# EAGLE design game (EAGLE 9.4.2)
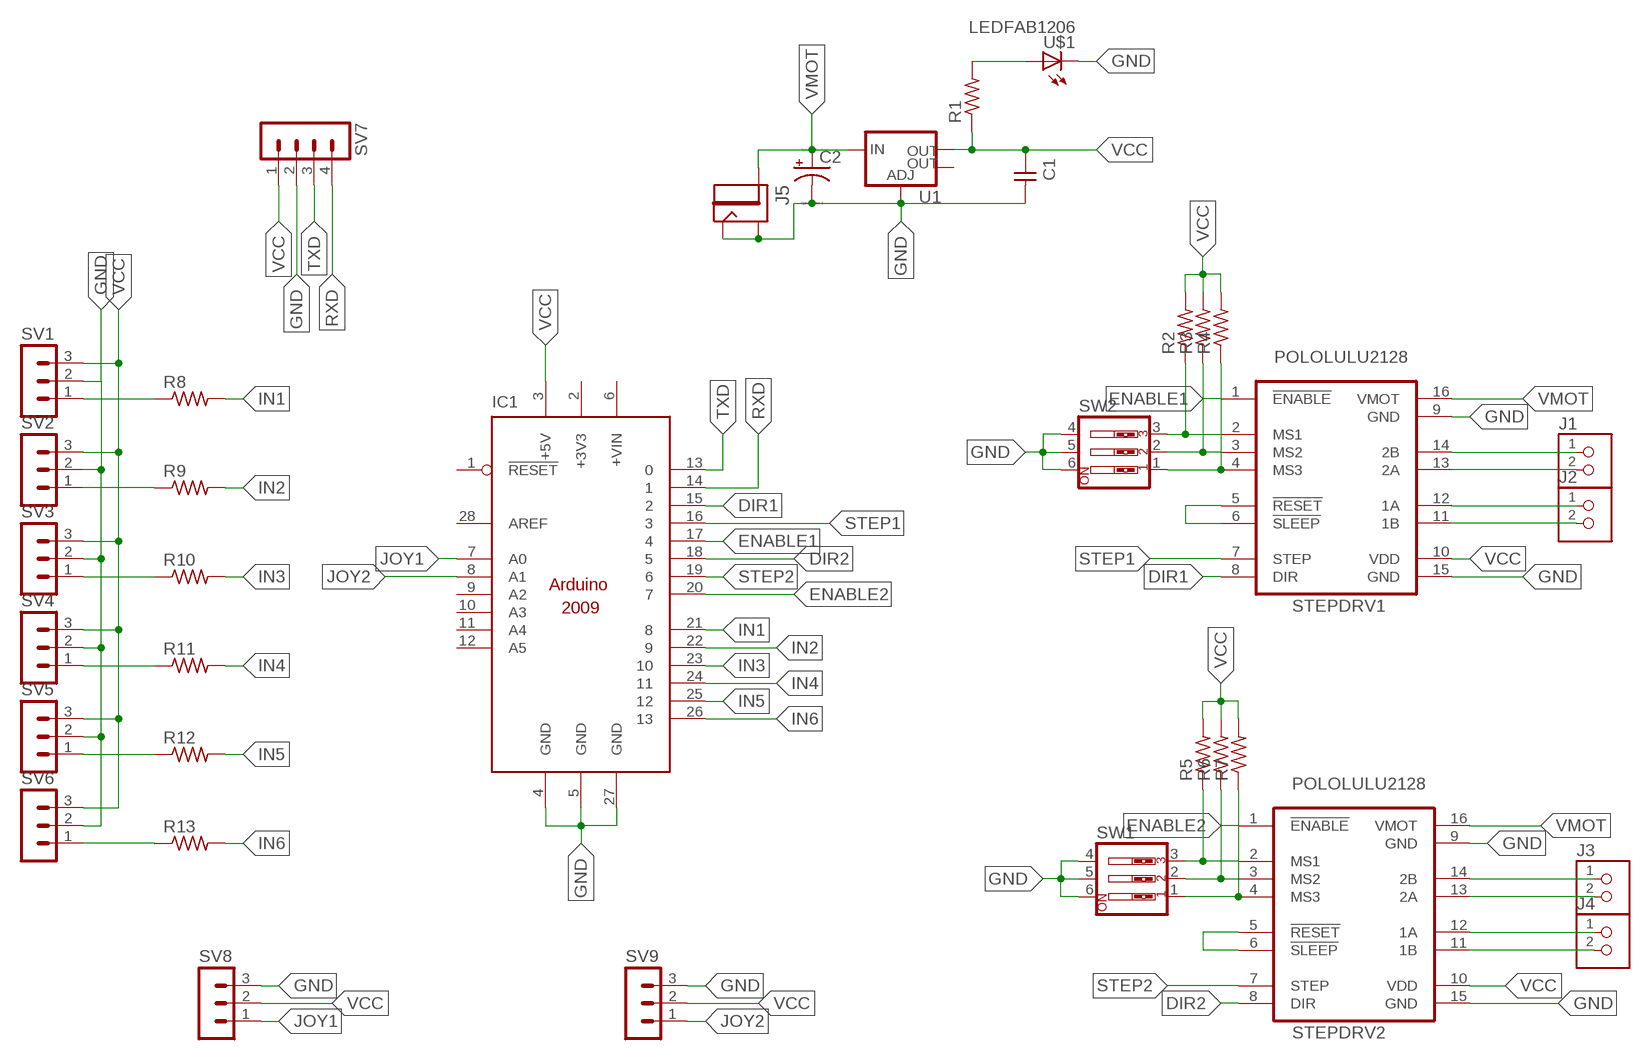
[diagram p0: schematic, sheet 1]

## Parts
C1  CAP-UNPOLARIZEDFAB  [C1206FAB]
C2  CPOL-USE1.8-4  [E1,8-4]
IC1  ARDUINO2009_10  [ARDUINO2009]
J1  TERM-1X02-ADAFRUIT  [3.5MMTERM]
J2  TERM-1X02-ADAFRUIT  [3.5MMTERM]
J3  TERM-1X02-ADAFRUIT  [3.5MMTERM]
J4  TERM-1X02-ADAFRUIT  [3.5MMTERM]
J5  JACK2.1MM  [JACK_2.1MM]
R1  RES-US1206FAB  [R1206FAB]
R2  RES-US1206FAB  [R1206FAB]
R3  RES-US1206FAB  [R1206FAB]
R4  RES-US1206FAB  [R1206FAB]
R5  RES-US1206FAB  [R1206FAB]
R6  RES-US1206FAB  [R1206FAB]
R7  RES-US1206FAB  [R1206FAB]
R8  RES-US1206FAB  [R1206FAB]
R9  RES-US1206FAB  [R1206FAB]
R10  RES-US1206FAB  [R1206FAB]
R11  RES-US1206FAB  [R1206FAB]
R12  RES-US1206FAB  [R1206FAB]
R13  RES-US1206FAB  [R1206FAB]
STEPDRV1  POLOLULU2128  [POLOLULU2128]
STEPDRV2  POLOLULU2128  [POLOLULU2128]
SV1  MA03-1  [MA03-1]
SV2  MA03-1  [MA03-1]
SV3  MA03-1  [MA03-1]
SV4  MA03-1  [MA03-1]
SV5  MA03-1  [MA03-1]
SV6  MA03-1  [MA03-1]
SV7  MA04-1  [MA04-1]
SV8  MA03-1  [MA03-1]
SV9  MA03-1  [MA03-1]
SW1  SW_DIP-3  [EDG-03]
SW2  SW_DIP-3  [EDG-03]
U1  V_REG_LM1117SOT223  [SOT223]
U$1  LEDFAB1206  [LED1206FAB]

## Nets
DIR1: IC1.15 STEPDRV1.8(DIR)
DIR2: IC1.18 STEPDRV2.8(DIR)
ENABLE1: IC1.17 STEPDRV1.1(!ENABLE)
ENABLE2: IC1.20 STEPDRV2.1(!ENABLE)
GND: C1.2 C2.- IC1.4(GND) IC1.5(GND) IC1.27(GND) J5.CONTACT J5.SHUNT STEPDRV1.9(GND) STEPDRV1.15(GND) STEPDRV2.9(GND) STEPDRV2.15(GND) SV1.2 SV2.2 SV3.2 SV4.2 SV5.2 SV6.2 SV7.2 SV8.3 SV9.3 SW1.4 SW1.5 SW1.6 SW2.4 SW2.5 SW2.6 U1.1(ADJ) U$1.2(C)
IN1: IC1.21 R8.2
IN2: IC1.22 R9.2
IN3: IC1.23 R10.2
IN4: IC1.24 R11.2
IN5: IC1.25 R12.2
IN6: IC1.26 R13.2
JOY1: IC1.7(A0) SV8.1
JOY2: IC1.8(A1) SV9.1
N$1: R2.1 STEPDRV1.2(MS1) SW2.3
N$2: STEPDRV1.5(!RESET) STEPDRV1.6(!SLEEP)
N$3: R8.1 SV1.1
N$4: R9.1 SV2.1
N$5: STEPDRV2.5(!RESET) STEPDRV2.6(!SLEEP)
N$6: R3.1 STEPDRV1.3(MS2) SW2.2
N$7: R4.1 STEPDRV1.4(MS3) SW2.1
N$9: J1.1 STEPDRV1.14(2B)
N$10: J1.2 STEPDRV1.13(2A)
N$11: J3.1 STEPDRV2.14(2B)
N$12: J3.2 STEPDRV2.13(2A)
N$13: J4.1 STEPDRV2.12(1A)
N$14: J4.2 STEPDRV2.11(1B)
N$15: R10.1 SV3.1
N$16: R11.1 SV4.1
N$17: J2.1 STEPDRV1.12(1A)
N$18: J2.2 STEPDRV1.11(1B)
N$19: R12.1 SV5.1
N$20: R13.1 SV6.1
N$24: R5.1 STEPDRV2.2(MS1) SW1.3
N$25: R6.1 STEPDRV2.3(MS2) SW1.2
N$26: R7.1 STEPDRV2.4(MS3) SW1.1
N$27: R1.2 U$1.1(A)
RXD: IC1.14 SV7.4
STEP1: IC1.16 STEPDRV1.7(STEP)
STEP2: IC1.19 STEPDRV2.7(STEP)
TXD: IC1.13 SV7.3
VCC: C1.1 IC1.3(+5V) R1.1 R2.2 R3.2 R4.2 R5.2 R6.2 R7.2 STEPDRV1.10(VDD) STEPDRV2.10(VDD) SV1.3 SV2.3 SV3.3 SV4.3 SV5.3 SV6.3 SV7.1 SV8.2 SV9.2 U1.2(OUT)
VMOT: C2.+ J5.PIN STEPDRV1.16(VMOT) STEPDRV2.16(VMOT) U1.3(IN)
Unconnected: IC1.1(!RESET) IC1.6(+VIN) IC1.9(A2) IC1.10(A3) IC1.11(A4) IC1.12(A5) IC1.28(AREF) U1.4(OUT)

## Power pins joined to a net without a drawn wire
+3V3: IC1.2(+3V3)

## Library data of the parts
C1 = fab:CAP-UNPOLARIZED
C2 = resistor:CPOL-US: POLARIZED CAPACITOR, American symbol
IC1 = arduino:ARDUINO2009_1: The Arduino Duemilanove ("2009") is a microcontroller board based on the ATmega168 or ATmega328. - 14 digital input/output pins (of which 6 can be used as PWM outputs) - 6 analog inputs, a 16 MHz crystal oscillator - USB connection - power jack - ISP header - reset button It contains everything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
J1-J4 = fab:TERM-1X02: 3.5mm terminal block, 2 positions ED555-2DS as found in the fablab inventory.
J5 = fab:JACK
R1-R13 = fab:RES-US: Resistor (US Symbol)
STEPDRV1 STEPDRV2 = stepper_drivers_etc:POLOLULU2128
SV1-SV6 SV8 SV9 = con-lstb:MA03-1: PIN HEADER; OC_FARNELL: unknown; OC_NEWARK: unknown
SV7 = con-lstb:MA04-1: PIN HEADER; OC_FARNELL: unknown; OC_NEWARK: unknown
SW1 SW2 = special:SW_DIP-3: DIP SWITCH
U1 = fab:V_REG_LM1117: Voltage Regulator LM1117 Standard adjustable voltage regulator but in SMD form. Spark Fun Electronics SKU : COM-00595; PROD_ID: VREG-08170
U$1 = fab:LED: LED

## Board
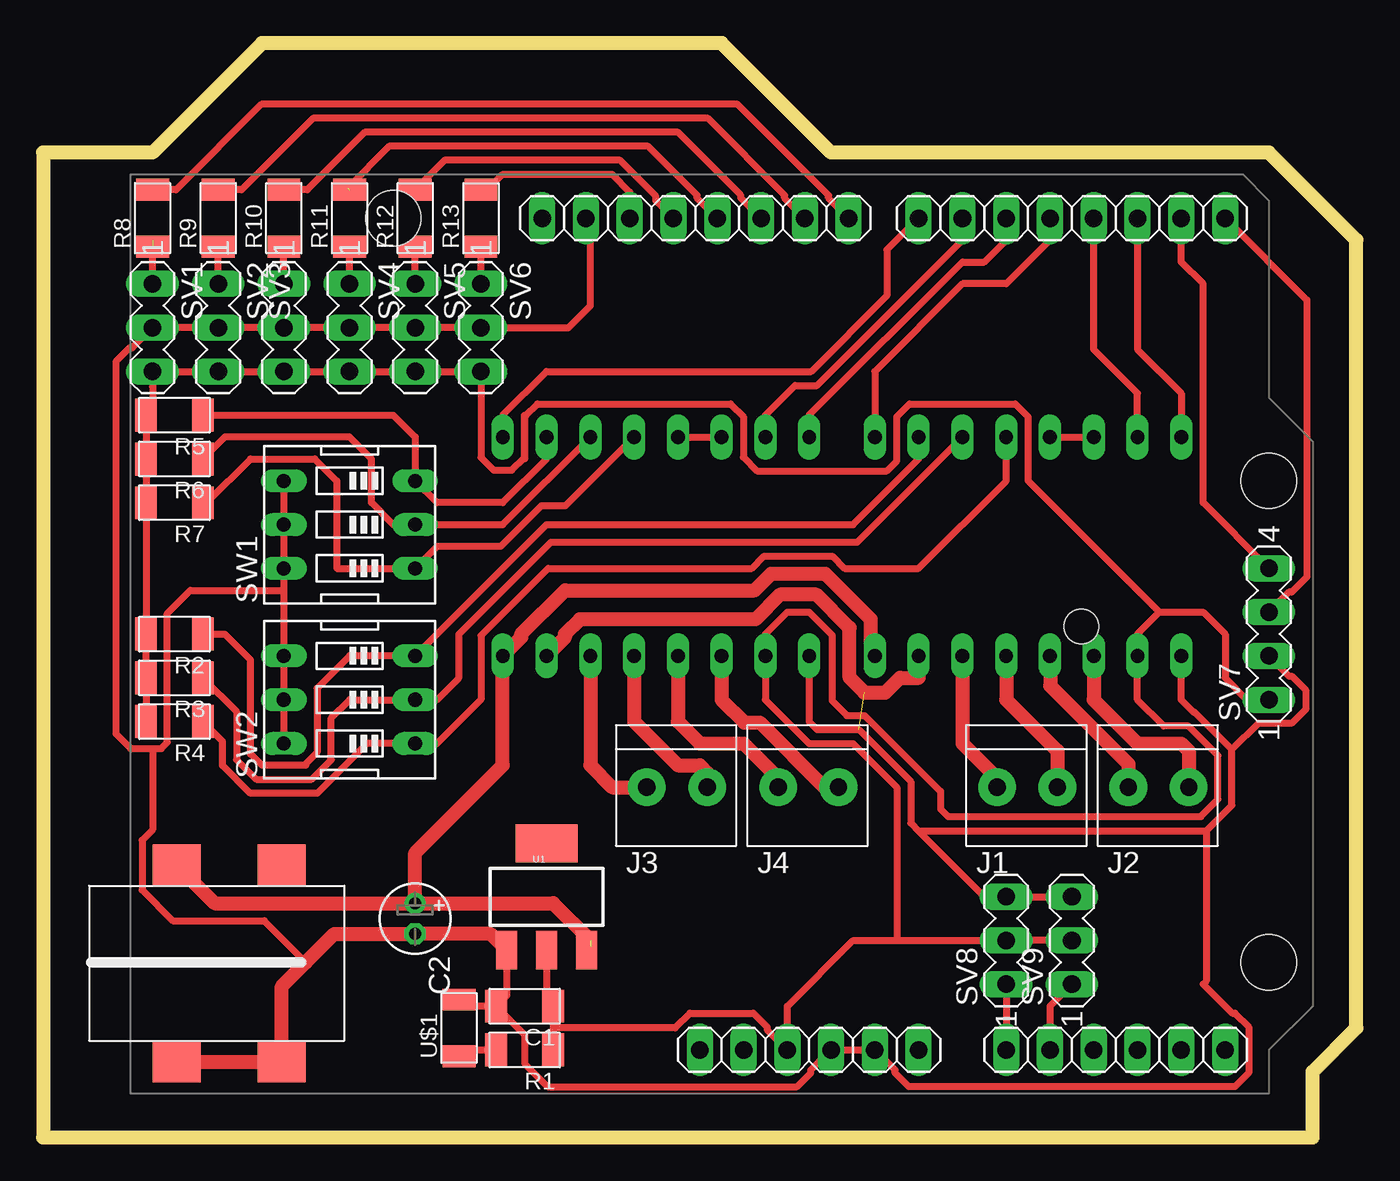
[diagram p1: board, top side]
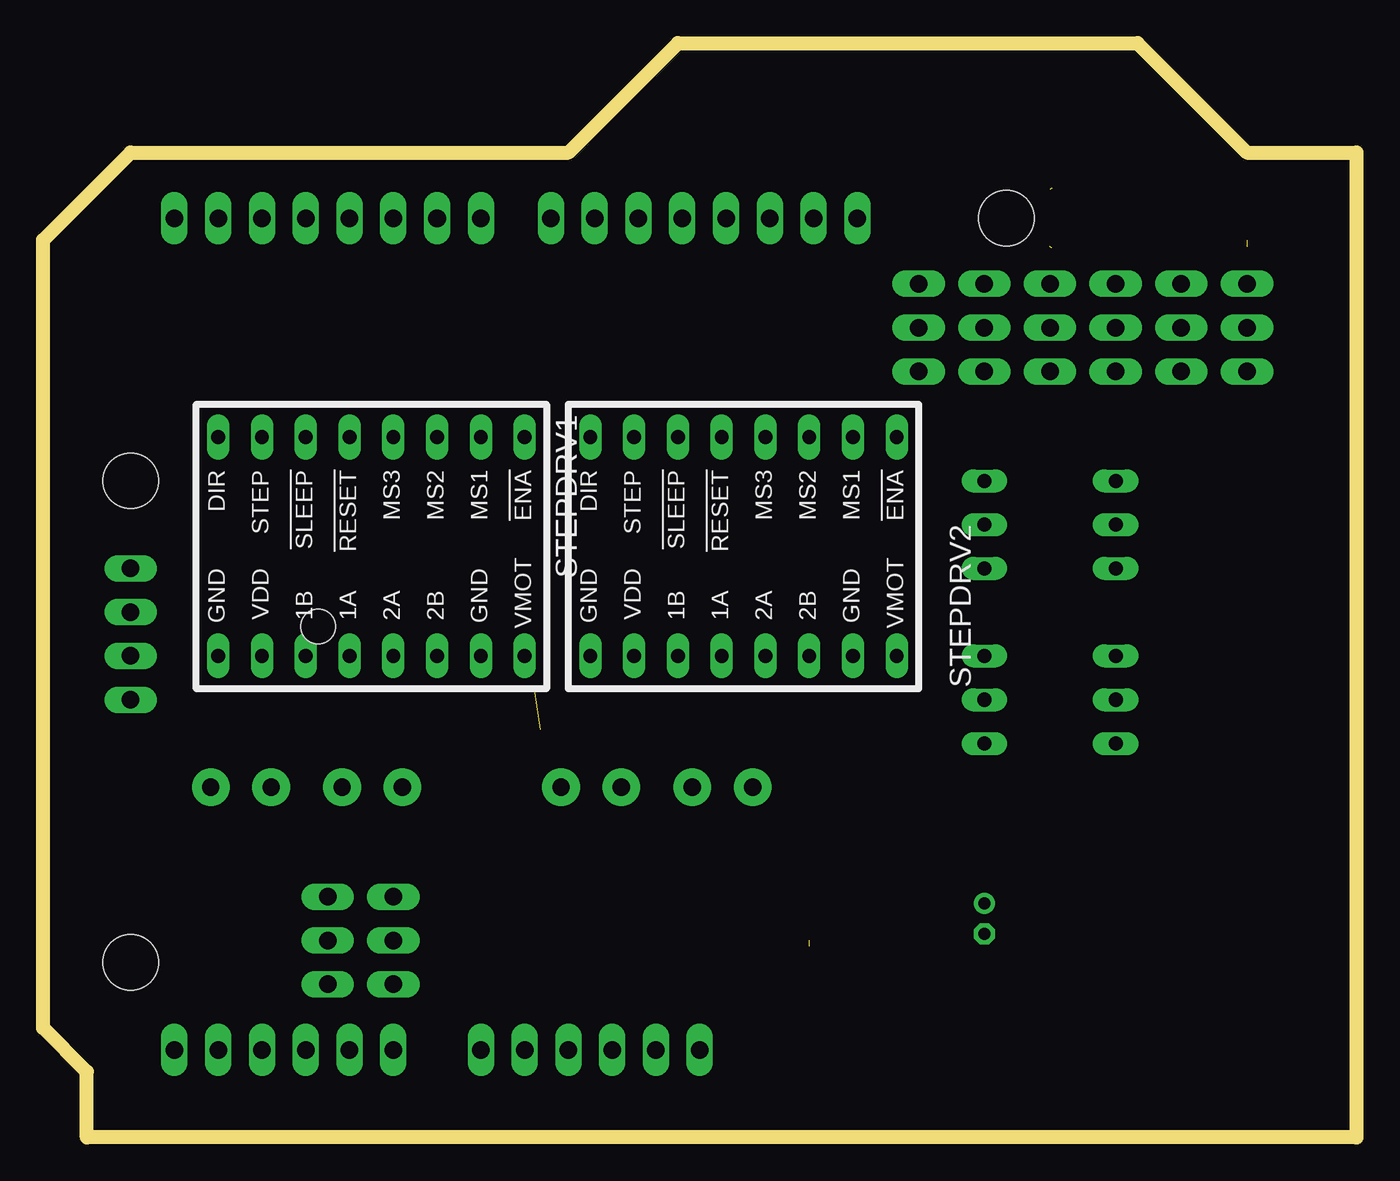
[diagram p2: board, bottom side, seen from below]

Size 76.2 x 63.5 mm. Coordinates in mm from the lower left corner, seen from the top.
Outline: 12.7,63.5 6.35,57.15 0,57.15 0,0 73.66,0 73.66,3.81 76.2,6.35 76.2,52.07 71.12,57.15 45.72,57.15 39.37,63.5 12.7,63.5
Copper layers (1*16): Top 0.035mm / dielectric 1.5mm / Bottom 0.035mm
Design rules "default *": minimum track width 16mil, minimum drill 0.35mm, track to track 16mil, track to pad 16mil, pad to pad 16mil, via to via 16mil, smd to smd 16mil, copper to edge 16mil, drill to drill 16mil, minimum pad ring 10mil, minimum via ring 8mil, stop-mask expansion 4mil, vias tented up to drill 0mil, thermal gap 10mil

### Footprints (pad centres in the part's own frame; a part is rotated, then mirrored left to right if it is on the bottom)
C1206FAB = smd 1.27 x 1.905: 1 -1.651,0; 2 1.651,0
E1,8-4 = drill 0.711 pad 1.168: + -0.889,0 | drill 0.711 pad 1.168 octagon: - 0.889,0
ARDUINO2009 = drill 1.016 long: 1 33.02,2.54; 2 35.56,2.54; 3 38.1,2.54; 4 40.64,2.54; 5 43.18,2.54; 6 45.72,2.54; 7 50.8,2.54; 8 53.34,2.54; 9 55.88,2.54; 10 58.42,2.54; 11 60.96,2.54; 12 63.5,2.54; 13 63.5,50.8; 14 60.96,50.8; 15 58.42,50.8; 16 55.88,50.8; 17 53.34,50.8; 18 50.8,50.8; 19 48.26,50.8; 20 45.72,50.8; 21 41.656,50.8; 22 39.116,50.8; 23 36.576,50.8; 24 34.036,50.8; 25 31.496,50.8; 26 28.956,50.8; 27 26.416,50.8; 28 23.876,50.8 | hole 3.2: 15.24,50.8; 66.04,35.56; 66.04,7.62 | hole 2: 55.17,27.114
3.5MMTERM = drill 1 pad 2.184: 1 1.8,0; 2 -1.7,0
JACK_2.1MM = smd 2.388 x 2.794: CONTACT 5.766,-2.413; PIN -5.639,-2.413; PIN1 -5.639,3.683; SHUNT 5.766,3.683
R1206FAB = smd 1.27 x 1.905: 1 -1.651,0; 2 1.651,0
POLOLULU2128 = drill 0.8 long: 1 -7.62,7.62; 2 -7.62,5.08; 3 -7.62,2.54; 4 -7.62,0; 5 -7.62,-2.54; 6 -7.62,-5.08; 7 -7.62,-7.62; 8 -7.62,-10.16; 9 5.08,-10.16; 10 5.08,-7.62; 11 5.08,-5.08; 12 5.08,-2.54; 13 5.08,0; 14 5.08,2.54; 15 5.08,5.08; 16 5.08,7.62
MA03-1 = drill 1.016 long: 1 -2.54,0; 2 0,0; 3 2.54,0
MA04-1 = drill 1.016 long: 1 -3.81,0; 2 -1.27,0; 3 1.27,0; 4 3.81,0
EDG-03 = drill 0.813 long: 1 -2.54,-3.81; 2 0,-3.81; 3 2.54,-3.81; 4 2.54,3.81; 5 0,3.81; 6 -2.54,3.81
SOT223 = smd 1.219 x 2.235: 1 -2.311,-3.099; 2 0,-3.099; 3 2.311,-3.099 | smd 3.6 x 2.2: 4 0,3.099
LED1206FAB = smd 1.27 x 1.905: 1 -1.651,0; 2 1.651,0

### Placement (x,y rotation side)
C1  27.94,7.62 180 top
C2  21.59,12.7 270 top
IC1  5.08,2.54 0 top
J1  57.15,20.32 180 top
J2  64.77,20.32 180 top
J3  36.83,20.32 180 top
J4  44.45,20.32 180 top
J5  10.16,10.16 270 top
R1  27.94,5.08 180 top
R2  7.62,29.21 180 top
R3  7.62,26.67 180 top
R4  7.62,24.13 180 top
R5  7.62,41.91 180 top
R6  7.62,39.37 180 top
R7  7.62,36.83 180 top
R8  6.35,53.34 90 top
R9  10.16,53.34 90 top
R10  13.97,53.34 90 top
R11  17.78,53.34 90 top
R12  21.59,53.34 90 top
R13  25.4,53.34 90 top
STEPDRV1  55.88,33.02 270 bottom
STEPDRV2  34.29,33.02 270 bottom
SV1  6.35,46.99 270 top
SV2  10.16,46.99 270 top
SV3  13.97,46.99 270 top
SV4  17.78,46.99 270 top
SV5  21.59,46.99 270 top
SV6  25.4,46.99 270 top
SV7  71.12,29.21 90 top
SV8  55.88,11.43 90 top
SV9  59.69,11.43 90 top
SW1  17.78,35.56 90 top
SW2  17.78,25.4 90 top
U1  29.21,13.97 0 top
U$1  24.13,6.35 90 top

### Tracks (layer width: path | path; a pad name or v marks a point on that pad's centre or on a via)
DIR1
  Top 0.406: STEPDRV1.8 66.04,43.18 63.5,45.72 IC1.15
DIR2
  Top 0.406: STEPDRV2.8 44.45,41.91 53.34,50.8 54.61,50.8 55.88,52.07 IC1.18
ENABLE1
  Top 0.406: IC1.17 58.42,52.07 55.88,49.53 53.34,49.53 48.26,44.45 STEPDRV1.1
ENABLE2
  Top 0.406: STEPDRV2.1 26.67,41.91 29.21,44.45 44.57,44.45 48.96,48.84 48.96,51.5 IC1.20
GND  (1 unrouted)
  Top 0.406: SV9.3 SV8.3 54.61,13.97 50.8,17.78 | 68.99,22.5 68.99,19.28 67.49,17.78 | 68.99,22.5 66.8,24.69 66.75,24.69 66.04,25.4 STEPDRV1.9 | U1.1 26.9,8.23 C1.2 | C1.2 24.51,7.62 U$1.2 | C1.2 27.94,5.97 27.94,4.28 29.27,2.95 43.75,2.95 44.55,3.75 44.55,3.91 IC1.4 IC1.5 49.43,3.91 49.43,3.75 50.23,2.95 69.15,2.95 69.95,3.75 69.95,6.41 69.15,7.21 68.99,7.21 67.31,8.89 67.49,9.07 67.49,17.78 | IC1.27 31.75,53.09 31.75,48.26 30.48,46.99 SV6.2 SV5.2 SV4.2 SV3.2 SV2.2 SV1.2 5.18,45.82 5.02,45.82 4.22,45.02 4.22,23.43 5.08,22.57 6.35,22.57 | 68.99,22.5 70.51,24.03 72.45,24.03 73.25,24.83 73.25,25.97 72.45,26.77 72.29,26.77 SV7.2 | 50.8,17.78 50.34,18.24 50.34,20.66 47.33,23.67 44.91,23.67 44.45,24.13 STEPDRV2.9 | 50.8,17.78 67.49,17.78 | SW1.4 SW1.6 | SW1.5 SW1.6 | SW2.6 SW2.5 SW2.4 13.97,31.75 | SW1.6 13.97,31.75 | 6.35,22.57 6.86,22.57 7.21,22.92 7.21,30.41 8.55,31.75 13.97,31.75 | 15.24,10.16 12.83,12.57 7.52,12.57 5.74,14.35 5.74,17.25 6.35,17.86 6.35,22.57
  Top 0.813: J5.CONTACT J5.SHUNT 13.84,8.76 15.24,10.16 16.89,11.81 C2.- 25.96,11.81 U1.1 | STEPDRV1.15 50.8,26.67 49.72,26.67 48.87,25.82 47.65,25.82 46.79,26.68 46.79,29.57 44.87,31.5 42.76,31.5 41.32,30.06 31.14,30.06 30.28,29.2 30.28,29.01 STEPDRV2.15
IN1
  Top 0.406: IC1.21 45.57,54.51 45.57,54.67 40.29,59.94 12.66,59.94 7.71,54.99 R8.2
IN2
  Top 0.406: IC1.22 43.03,54.51 43.03,54.67 38.57,59.13 15.66,59.13 11.52,54.99 R9.2
IN3
  Top 0.406: IC1.23 40.49,54.51 40.49,54.67 36.84,58.32 18.66,58.32 15.33,54.99 R10.2
IN4  (1 unrouted)
  Top 0.406: IC1.24 37.95,54.51 37.95,54.67 35.11,57.51 20.09,57.51 17.68,55.09
IN5
  Top 0.406: IC1.25 35.56,54.36 35.56,54.61 33.48,56.69 23.29,56.69 R12.2
IN6
  Top 0.406: R13.2 25.78,54.99 26.67,55.88 33.02,55.88 34.04,54.86 IC1.26
JOY1
  Top 0.406: SV8.1 IC1.7
JOY2
  Top 0.406: SV9.1 58.42,7.62 IC1.8
N$1
  Top 0.406: 8.89,29.21 R2.1 10.54,29.21 12.04,27.71 12.04,22.25 12.7,21.59 15.24,21.59 15.24,21.67 15.9,22.33 15.9,26.06 17.78,27.94 SW2.3 29.21,35.56 46.99,35.56 50.8,39.37 STEPDRV1.2
N$2
  Top 0.406: STEPDRV1.5 STEPDRV1.6
N$3  (1 unrouted)
  Top 0.406: SV1.1 6.35,52.07
N$4
  Top 0.406: SV2.1 R9.1
N$5
  Top 0.406: STEPDRV2.5 STEPDRV2.6
N$6
  Top 0.406: 9.27,26.58 R3.1 11.23,24.71 11.23,21.91 12.36,20.78 15.58,20.78 16.71,21.91 16.71,24.33 17.78,25.4 SW2.2 22.86,25.4 24.13,26.67 24.13,29.21 29.46,34.54 47.24,34.54 STEPDRV1.3
N$7
  Top 0.406: STEPDRV1.4 55.88,38.1 50.8,33.02 46.51,33.02 45.8,33.73 41.83,33.73 41.12,33.02 29.31,33.02 25.41,29.12 25.41,25.41 22.86,22.86 SW2.1 18.81,22.86 15.91,19.96 12.03,19.96 10.41,21.58 10.41,22.99 R4.1
N$9
  Top 0.813: J1.1 55.35,20.85 53.34,22.86 STEPDRV1.14
N$10
  Top 0.813: J1.2 58.85,22.43 55.88,25.4 STEPDRV1.13
N$11
  Top 0.813: STEPDRV2.14 31.75,21.59 33.02,20.32 J3.1
N$12
  Top 0.813: STEPDRV2.13 34.29,24.13 36.83,21.59 38.1,21.59 38.53,21.16 J3.2
N$13
  Top 0.813: STEPDRV2.12 36.83,24.13 38.1,22.86 40.64,22.86 42.65,20.85 J4.1
N$14
  Top 0.813: STEPDRV2.11 39.37,25.4 40.69,24.08 41.59,24.08 45.34,20.32 J4.2
N$15
  Top 0.406: SV3.1 R10.1
N$16  (1 unrouted)
  Top 0.406: SV4.1 17.78,51.48 17.68,51.59 17.34,51.24
N$17
  Top 0.813: J2.1 62.97,21.67 58.44,26.2 58.44,27.92 STEPDRV1.12
N$18
  Top 0.813: STEPDRV1.11 60.96,25.4 63.5,22.86 66.04,22.86 66.47,22.43 J2.2
N$19
  Top 0.406: SV5.1 R12.1
N$20
  Top 0.406: SV6.1 R13.1
N$24
  Top 0.406: R5.1 20.32,41.91 21.59,40.64 SW1.3 22.86,36.83 26.67,36.83 29.21,39.37 STEPDRV2.2
N$25
  Top 0.406: R6.1 10.54,40.64 17.78,40.64 19.05,39.37 19.05,36.83 20.32,35.56 SW1.2 26.67,35.56 STEPDRV2.3
N$26
  Top 0.406: R7.1 9.5,36.83 12.04,39.37 15.77,39.37 17.04,38.1 17.04,33.02 SW1.1 22.86,34.29 26.55,34.29 28.9,36.64 30.29,36.64 STEPDRV2.4
N$27
  Top 0.406: U$1.1 24.51,5.08 R1.2
RXD
  Top 0.406: SV7.4 67.31,36.83 67.31,49.53 66.04,50.8 IC1.14
STEP1
  Top 0.406: STEPDRV1.7 63.5,43.18 60.96,45.72 IC1.16
STEP2
  Top 0.406: STEPDRV2.7 41.91,41.91 43.64,43.64 44.91,43.64 53.34,52.07 IC1.19
TXD
  Top 0.406: SV7.3 72.29,31.65 72.45,31.65 73.33,32.53 73.33,48.59 IC1.13
VCC
  Top 0.406: R4.2 R3.2 R2.2 R7.2 R6.2 R5.2 6.35,42.29 SV1.3 | SV9.2 SV8.2 49.53,11.43 | 49.53,11.43 46.99,11.43 43.18,7.62 IC1.3 42.01,6.25 42.01,6.41 41.21,7.21 37.53,7.21 36.67,6.35 29.59,6.35 | U1.2 29.21,7.62 C1.1 29.59,6.35 | 29.59,6.35 R1.1 | SV1.3 SV2.3 SV3.3 SV4.3 SV5.3 SV6.3 25.41,39.46 26.15,38.72 27.19,38.72 27.93,39.46 27.93,41.9 | SV1.3 6.35,43.56 | 64.77,30.48 63.5,29.21 STEPDRV1.10 63.5,25.4 65.02,23.88 66.46,23.88 68.17,22.16 68.17,19.62 67.18,18.62 52.5,18.62 52.07,19.05 52.07,20.08 47.66,24.49 46.63,24.49 45.78,25.34 45.78,29.15 44.45,30.48 43.18,30.48 41.91,29.21 STEPDRV2.10 41.91,25.4 44.45,22.86 46.99,22.86 49.53,20.32 49.53,11.43 | 64.77,30.48 67.31,30.48 68.58,29.21 68.58,26.67 69.85,25.4 SV7.1 | 27.94,39.37 27.94,41.91 27.93,41.9 | 27.93,41.9 28.03,41.9 28.69,42.56 39.89,42.56 40.63,41.82 40.63,39.48 41.43,38.67 48.96,38.67 49.54,39.26 49.54,41.82 50.28,42.56 56.4,42.56 57.14,41.82 57.14,38.11 64.77,30.48
VMOT  (1 unrouted)
  Top 0.813: J5.PIN 9.96,13.59 C2.+ | 31.75,11.1 U1.3 | C2.+ 21.59,16.51 26.67,21.59 STEPDRV2.16 27.74,29.01 27.74,29.2 30.29,31.75 41.29,31.75 42.25,32.72 45.38,32.72 48.01,30.08 48.01,28.19 STEPDRV1.16 | C2.+ 29.59,13.59 31.75,11.43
